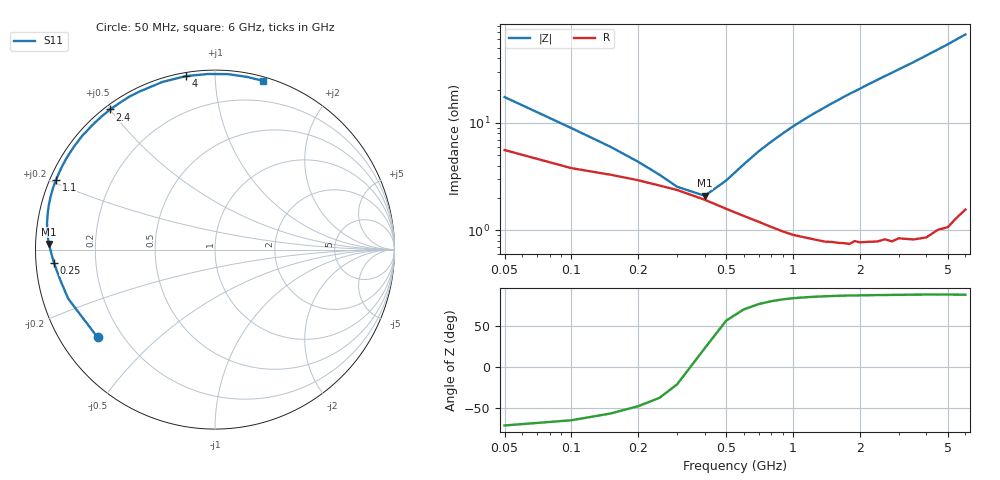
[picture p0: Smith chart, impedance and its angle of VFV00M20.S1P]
! Infineon Technologies  Discrete & RF Semiconductors
! BBY 58-03
! Si Tuning Diode in SOD323
! VR =
! S-Parameters:  June  1999
# GHz  S  MA  R  50
!  f  S11
! GHz  MAG  ANG
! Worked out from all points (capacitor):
!   34 points, 50 MHz to 6 GHz, reference 50 ohm
!   read as one part to ground: C = 181 pF near 50 MHz
!   lowest |Z| = 2.1 ohm at 400 MHz (marker M1)
!   series resonance near 352.5 MHz, so ESL is about 1.1 nH
!   S11 on the Smith chart (normalised r, x): 50 MHz: 0.11, -0.33; 250 MHz: 0.05, -0.04; 1.1 GHz: 0.02, +0.21; 2.4 GHz: 0.02, +0.50; 4 GHz: 0.02, +0.85; 6 GHz: 0.03, +1.33
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0.05  0.817 -143.2
0.1  0.8623 -161.5
0.15  0.8775 -168.5
0.2  0.8898 -172.6
0.25  0.9008 -175.4
0.3  0.9092 -177.9
0.4  0.9258 178.1
0.5  0.9386 174.4
0.6  0.9473 171.1
0.8  0.9587 164.9
1  0.9654 159.1
1.1  0.9671 156.4
1.2  0.9687 153.7
1.4  0.9713 148.7
1.6  0.9727 143.9
1.8  0.974 139.2
2  0.9739 135.0
2.2  0.9744 130.7
2.4  0.9751 126.8
2.6  0.9748 122.9
2.8  0.9767 119.3
3  0.9761 115.7
3.5  0.9788 107.5
4  0.9801 99.5
4.5  0.9792 92.3
5  0.9803 85.8
5.5  0.9786 79.5
6  0.9776 74.0
